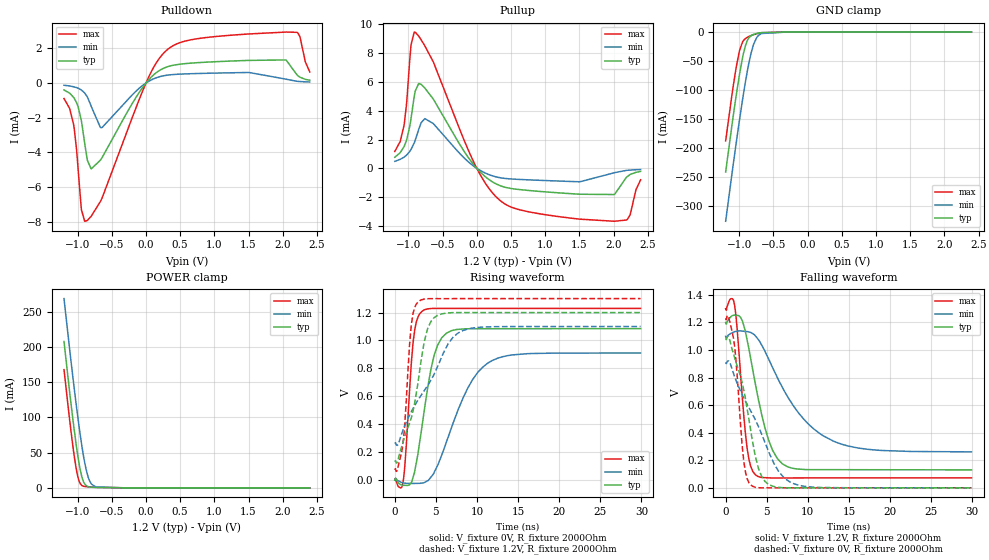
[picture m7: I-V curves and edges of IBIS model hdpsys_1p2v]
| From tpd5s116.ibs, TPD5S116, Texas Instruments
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[Model]   hdpsys_1p2v
Model_type   3-state
Polarity   Non-Inverting
Vmeas = 0.6
Vref = 1.2
Cref = 15pF
Rref = 2000
|   typ   min   max
|   (fast PVT)   (slow PVT)   (nom PVT)
C_comp   1.1241p   1.0342p   1.3025p
|C_comp (High state)   1.1241p   1.0342p   1.3025p
|C_comp (Low state)   1.0197p   0.970p   1.0858p
| Where nom  PVT is Nominal Process, 1.2V, 27C
|   Fast PVT is Strong Process,  1.3V, -40C
|   Slow PVT is Weak Process,   1.1V, 125C
[Voltage Range]   1.2   1.1   1.3
[Temperature Range]   27   125   -40
[Pullup Reference]   1.2   1.1   1.3
[Pulldown Reference]   -0   -0   -0
[Power Clamp Reference]   1.2   1.1   1.3
[GND Clamp Reference]   -0   -0   -0
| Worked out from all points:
|   slope of the pulldown table from 0 to 0.18 V, typ, clamps not added: 264 ohm
|   slope of the pullup table from 0 to 0.18 V, typ, clamps not added: 230 ohm
|   POWER clamp passes 1 mA (typ) near -0.81 V on its own axis
|   falling waveform, V_fixture 1.2V, R_fixture 2000Ohm: 20-80 % time 2.34ns typ, 5.44ns min, 1.03ns max; typ from 1.2 V to 0.13 V
|   rising waveform, V_fixture 0V, R_fixture 2000Ohm: 20-80 % time 1.8ns typ, 3.84ns min, 828ps max; typ from 0 V to 1.08 V
|   rising waveform, V_fixture 1.2V, R_fixture 2000Ohm: 20-80 % time 2.16ns typ, 4.6ns min, 823ps max; typ from 0.13 V to 1.2 V
|   falling waveform, V_fixture 0V, R_fixture 2000Ohm: 20-80 % time 2.17ns typ, 4.21ns min, 949ps max; typ from 1.08 V to 0 V
[Pulldown]
|   Voltage   I(typ)   I(min)   I(max)
-1.2V     -401.9uA   -129.3uA   -896.7uA
-1.06V    -826uA     -217.5uA   -2.392mA
-1.016V   -1.133mA   -267.7uA   -3.824mA
-948mV    -2.125mA   -398.8uA   -7.201mA
-894mV    -3.57mA    -590.9uA   -7.98mA
-804mV    -4.947mA   -1.316mA   -7.697mA
-642mV    -4.303mA   -2.567mA   -6.632mA
6mV       29.6uA     15.46uA    54.9uA
355.2mV   984.2uA    472.4uA    2.054mA
2.047V    1.329mA    223uA      2.94mA
2.209V    468.1uA    98.87uA    2.923mA
2.396V    158.6uA    56.89uA    634.5uA
[GND Clamp]
|   Voltage   I(typ)   I(min)   I(max)
-1.2V     -240.8mA   -325.6mA   -187.2mA
-1.085V   -140.9mA   -224.1mA   -89.72mA
-1.042V   -106mA     -187.4mA   -58.08mA
-994.8mV  -71.11mA   -149.1mA   -31.06mA
-940.8mV  -37.49mA   -107.4mA   -14.77mA
-883.2mV  -14.75mA   -67.42mA   -9.063mA
-832.8mV  -6.617mA   -38.63mA   -6.306mA
-796.8mV  -4.241mA   -23.15mA   -4.698mA
-717.6mV  -1.8mA     -5.631mA   -2.018mA
-674.4mV  -1.054mA   -2.515mA   -1.084mA
-300mV    -296nA     -2.806uA   -30.92nA
2.396V    0A         0A         0A
[Pullup]
|   Voltage   I(typ)   I(min)   I(max)
-1.2V     771.5uA    488uA      1.176mA
-1.067V   1.491mA    774.6uA    2.953mA
-1.027V   1.977mA    926.5uA    4.556mA
-962.4mV  3.478mA    1.317mA    8.593mA
-912mV    5.114mA    1.824mA    9.471mA
-850.8mV  5.891mA    2.705mA    9.19mA
-760.8mV  5.58mA     3.457mA    8.51mA
-4.8mV    25.7uA     14.68uA    45.02uA
405.6mV   -1.301mA   -695.5uA   -2.455mA
2.011V    -1.818mA   -305.3uA   -3.675mA
2.188V    -628uA     -140.3uA   -3.587mA
2.396V    -210uA     -81.5uA    -795.3uA
[POWER Clamp]
|   Voltage   I(typ)   I(min)   I(max)
-1.2V     207.5mA    268.4mA    167.6mA
-1.074V   100.6mA    160.3mA    62.22mA
-1.049V   81.07mA    139.8mA    44.25mA
-1.006V   50.49mA    106.2mA    19.31mA
-966mV    27.41mA    77.57mA    6.644mA
-915.6mV  8.903mA    45.69mA    2.292mA
-876mV    3.18mA     25.99mA    1.628mA
-847.2mV  1.699mA    15.54mA    1.387mA
-796.8mV  858.6uA    5.225mA    1.061mA
-735.6mV  518.5uA    1.294mA    721.7uA
-300mV    127.1nA    748.5nA    28.29nA
2.396V    0A         0A         0A
[Ramp]
R_load = 2000
|   typ   min   max
dV/dt_r   0.650798/1.79668e-09   0.546032/3.83789e-09   0.737841/8.28347e-10
dV/dt_f   0.641821/2.34476e-09   0.503441/5.4429e-09   0.73664/1.02598e-09
[Falling Waveform]
V_fixture = 1.2V
V_fixture_min = 1.1V
V_fixture_max = 1.3V
R_fixture = 2000Ohm
C_fixture = 0F
|   Time   V(typ)   V(min)   V(max)
0s        1.2V       1.1V       1.3V
1.082ns   1.254V     1.134V     1.329V
2.053ns   1.209V     1.137V     635.7mV
2.627ns   1.069V     1.134V     280.8mV
3.622ns   751.5mV    1.102V     93.71mV
5.695ns   273.8mV    874.7mV    71.63mV
7.495ns   153.6mV    665.7mV    71.67mV
10.68ns   131.8mV    429.1mV    71.76mV
14.28ns   131.5mV    313.4mV    71.85mV
29.9ns    130.3mV    260.9mV    72.27mV
[Rising Waveform]
V_fixture = 0V
V_fixture_min = 0V
V_fixture_max = 0V
R_fixture = 2000Ohm
C_fixture = 0F
|   Time   V(typ)   V(min)   V(max)
0s        5.044nV    302.1nV    1.357nV
949.7ps   -37.47mV   -20.07mV   -34.51mV
1.215ns   -38.93mV   -23.25mV   98.45mV
2.212ns   17.2mV     -25.43mV   980.2mV
3.303ns   383.5mV    -22.77mV   1.209V
4.792ns   895.5mV    54.24mV    1.23V
6.895ns   1.07V      375mV      1.23V
9.483ns   1.084V     721.1mV    1.23V
12.48ns   1.084V     872mV      1.23V
29.9ns    1.085V     910.1mV    1.23V
[Rising Waveform]
V_fixture = 1.2V
V_fixture_min = 1.1V
V_fixture_max = 1.3V
R_fixture = 2000Ohm
C_fixture = 0F
|   Time   V(typ)   V(min)   V(max)
0s        130.3mV    260.5mV    72.27mV
329.3ps   131.2mV    250mV      80.32mV
1.082ns   286.6mV    370.1mV    308.4mV
2.005ns   445.8mV    488.6mV    1.112V
3.042ns   791.8mV    593mV      1.286V
3.588ns   993.6mV    640.8mV    1.297V
4.391ns   1.136V     715.6mV    1.3V
6.483ns   1.197V     975.6mV    1.3V
8.283ns   1.2V       1.071V     1.3V
29.9ns    1.2V       1.1V       1.3V
[Falling Waveform]
|Gnd
V_fixture = 0V
V_fixture_min = 0V
V_fixture_max = 0V
R_fixture = 2000Ohm
C_fixture = 0F
|   Time   V(typ)   V(min)   V(max)
0s        1.085V     910.2mV    1.23V
329.3ps   1.095V     920.5mV    1.245V
1.082ns   946.4mV    808mV      1.03V
2.005ns   764.5mV    677.5mV    308.2mV
2.419ns   643.7mV    627.2mV    110.2mV
3.303ns   326.5mV    529.1mV    10.1mV
4.792ns   45.77mV    328.1mV    -174.2uV
6.483ns   3.232mV    115.5mV    -162.5uV
8.283ns   148.7uV    29.7mV     -150uV
29.9ns    7.568uV    67.24uV    75.53nV
